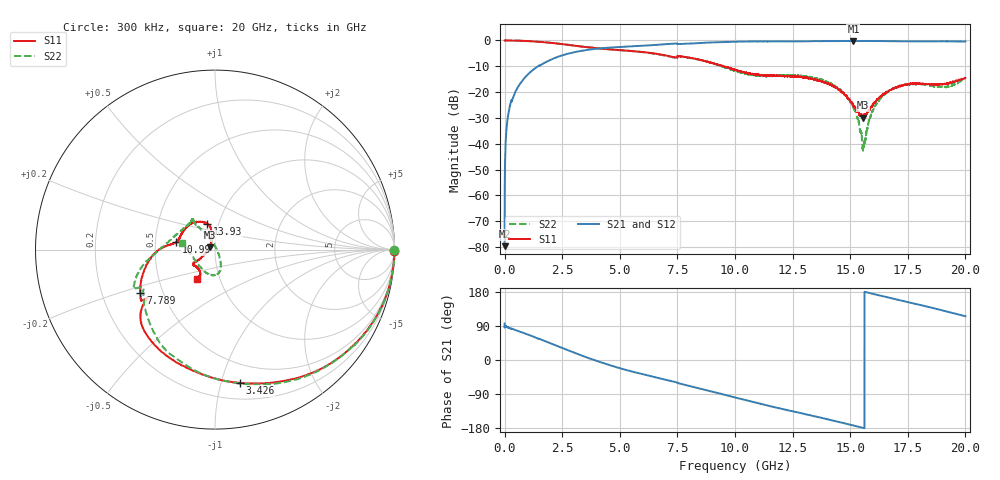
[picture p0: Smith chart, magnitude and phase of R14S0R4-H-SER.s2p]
!{R14S0R4}
!Johanson Technology Inc.
!www.johansontechnology.com
!Test Board Conditions:
!Substrate Type  RO4350B
!Substrate Thickness  20 mil
!Substrate Dk  3.66
!TL Type: GCPW
!TL Trace Width  36 mil
!TL Gap  12 mil
!Electrode orientation  Horizontal
!DUT TOPOLOGY	SERIES
!Mounting Pad LxW  26x36 mil
! Created Wed Nov 25 17:33:21 2020
! 2 Port Network Data from SP1.SP block
! freq  magS11  angS11  magS21  angS21  magS12  angS12  magS22  angS22
# khz S ma R 50
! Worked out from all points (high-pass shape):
!   20001 points, 300 kHz to 20 GHz, reference 50 ohm
!   highest |S21| = -0.19 dB at 15.14 GHz (marker M1); lowest = -79.6 dB at 300 kHz (marker M2)
!   |S21| within 3 dB of the highest: 3.987253 GHz to 3.987321 GHz (67.84 kHz wide, 0.0017 % of centre); 3.993 GHz to end of sweep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
!   lowest |S11| = -29.8 dB at 15.55 GHz (marker M3), VSWR 1.07, Z = 47.1 + j1.2 ohm
!   |S11| at or under -10 dB: 9.499 GHz to end of sweep
!   |S22| runs from -43.1 to 0.0 dB; largest |S21 - S12| = 0.011
!   S11 on the Smith chart (normalised r, x): 300 kHz: open; 3.426 GHz: 0.33, -1.15; 7.789 GHz: 0.37, -0.23; 10.99 GHz: 0.64, +0.06; 13.93 GHz: 0.88, +0.26; 20 GHz: 0.78, -0.26
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300  0.9971 -0.4  0.0001042 96.2  6.245e-05 85.7  0.9975 -0.2
102300  0.9996 -2.5  0.02418 87.3  0.02433 87.2  0.9994 -2.4
138300  0.9994 -3.3  0.03271 86.4  0.03285 86.6  0.999 -3.3
267300  0.9975 -6.5  0.06321 82.9  0.06348 82.9  0.9971 -6.5
520300  0.9929 -11.5  0.1125 78.1  0.1128 78.2  0.9931 -11.5
1407300  0.9464 -32.2  0.3076 57.7  0.3084 57.5  0.949 -32.3
3334300  0.7633 -77.3  0.6293 12.1  0.6302 12.1  0.7632 -78.3
3426300  0.7553 -79.5  0.6392 9.9  0.6404 9.9  0.7554 -80.3
5110300  0.6445 -116.7  0.7515 -23.5  0.7521 -23.4  0.6429 -110.0
6667300  0.5441 -139.6  0.8266 -47.4  0.8288 -47.3  0.5371 -133.9
7789300  0.4815 -149.8  0.8614 -65.0  0.8641 -65.1  0.4806 -158.3
1.00003e7  0.2711 175.4  0.9455 -98.8  0.9481 -98.9  0.26 169.0
1.09853e7  0.2188 168.7  0.96 -113.8  0.9593 -114.0  0.2075 143.0
1.33343e7  0.1801 120.5  0.9661 -146.9  0.9638 -146.9  0.1907 127.3
1.39333e7  0.1514 107.3  0.9733 -155.3  0.9667 -155.3  0.1627 126.1
1.46523e7  0.0998 99.2  0.9749 -165.7  0.9755 -165.6  0.1008 120.0
1.51423e7  0.05332 110.6  0.9787 -172.9  0.9756 -172.9  0.05021 111.9
1.55543e7  0.0322 156.8  0.975 -179.0  0.9767 -179.0  0.007894 37.6
1.60173e7  0.06025 -158.3  0.9743 174.1  0.9744 174.1  0.0472 -57.1
1.66673e7  0.1045 -149.1  0.9694 164.7  0.9678 164.7  0.1034 -71.6
1.92163e7  0.1485 -124.8  0.9647 127.5  0.9633 127.8  0.13 -156.0
2e7  0.1884 -121.5  0.9542 115.5  0.9457 115.3  0.1878 169.6
